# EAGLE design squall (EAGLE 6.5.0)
AUTHOR: Brad Campbell; REV: A; TITLE: Squall

## Sheet 1 of 2: nRF51822
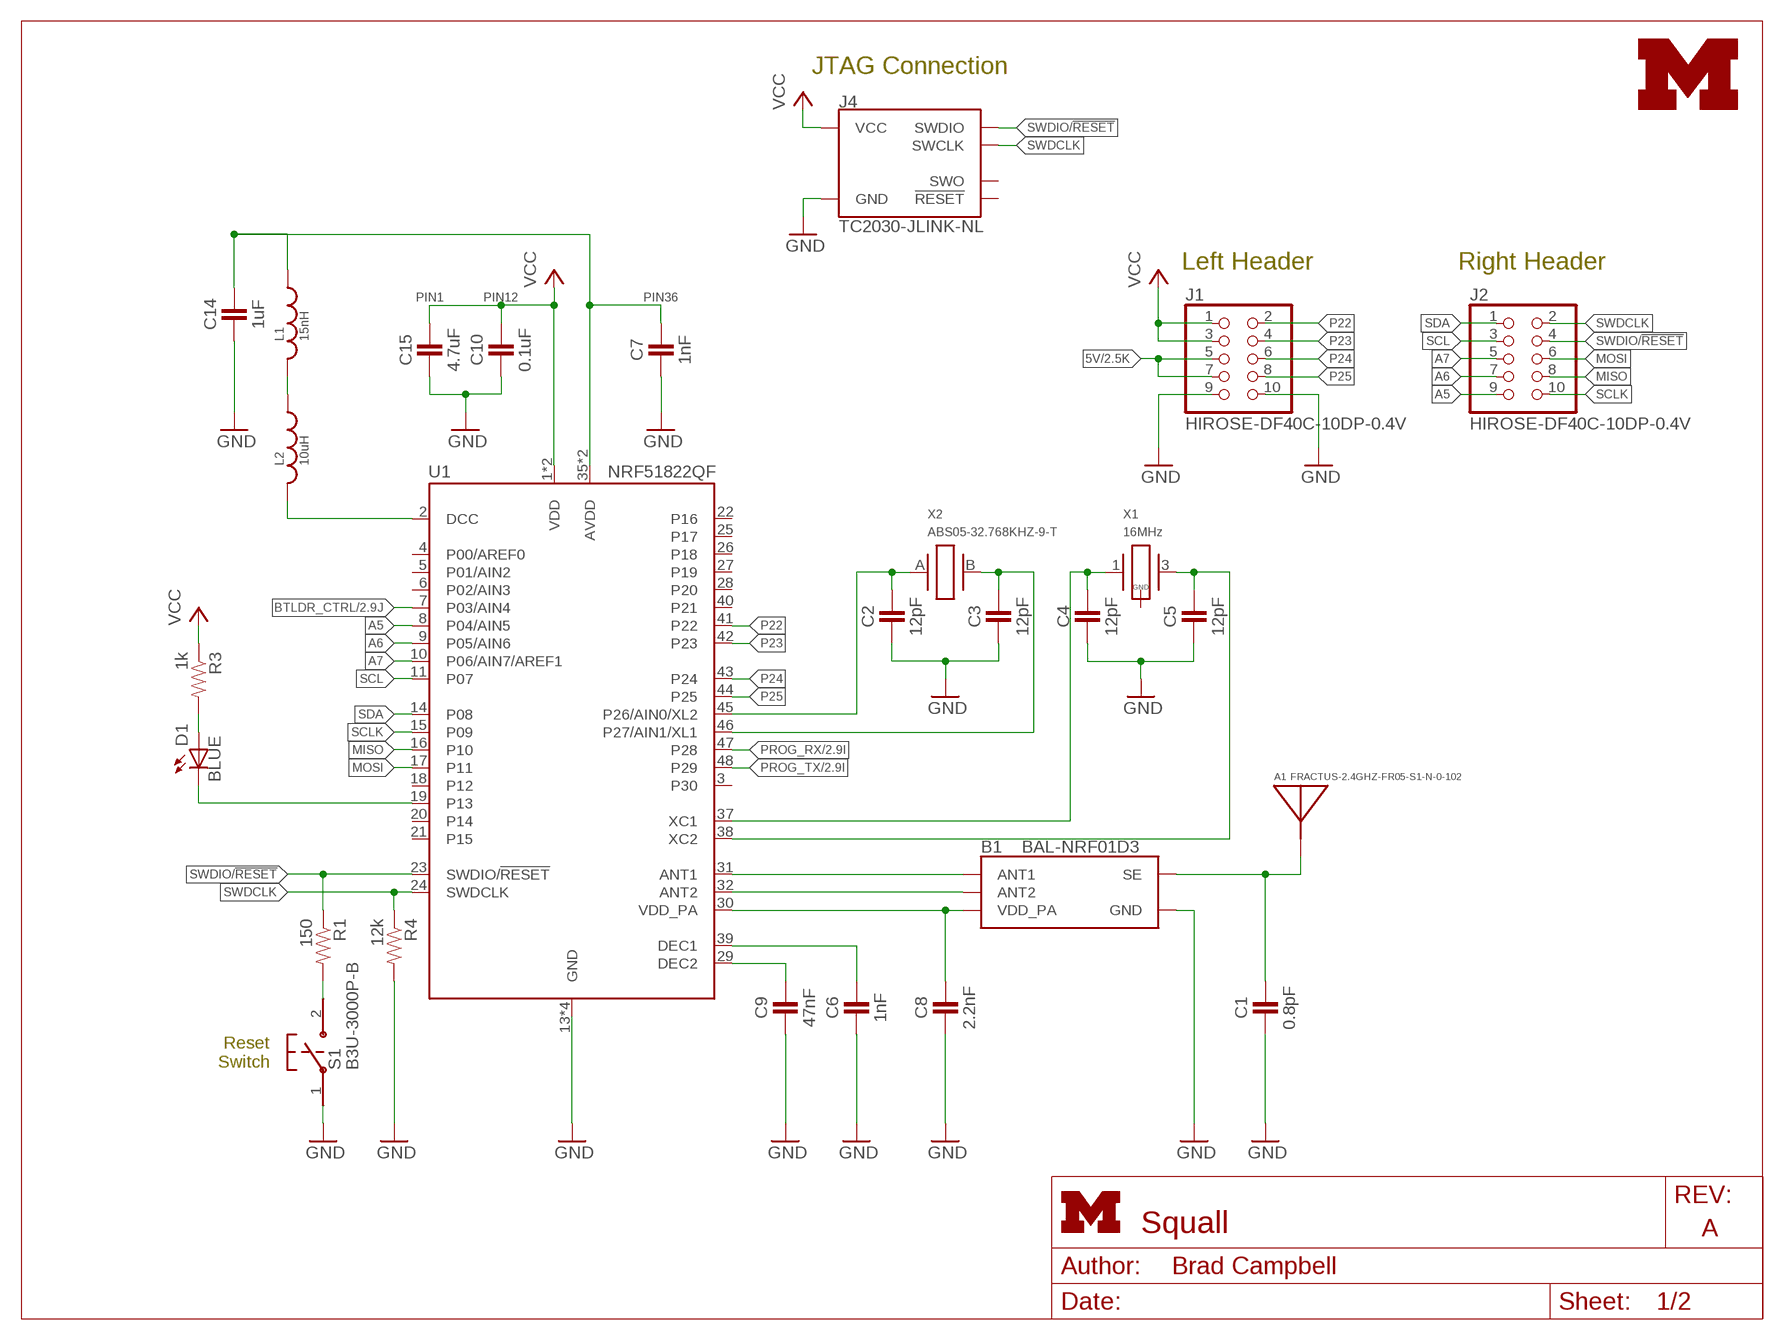
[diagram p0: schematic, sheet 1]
FRAME1 (LETTER_L): HEIGHT: 8.5in; WIDTH: 11in

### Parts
A1  FRACTUS-2.4GHZ-FR05-S1-N-0-102  [FRACTUS-ANTENNA-FR05-S1-N-0-102]
B1  BAL-NRF01D3  [BAL-NRF01D3]
C1  0.8pF  CAPACITOR  [0402_CAP]
C2  12pF  CAPACITOR  [0402_CAP]
C3  12pF  CAPACITOR  [0402_CAP]
C4  12pF  CAPACITOR  [0402_CAP]
C5  12pF  CAPACITOR  [0402_CAP]
C6  1nF  CAPACITOR  [0402_CAP]
C7  1nF  CAPACITOR  [0402_CAP]
C8  2.2nF  CAPACITOR  [0402_CAP]
C9  47nF  CAPACITOR  [0402_CAP]
C10  0.1uF  CAPACITOR  [0402_CAP]
C14  1uF  CAPACITOR  [0402_CAP]
C15  4.7uF  CAPACITOR  [0402_CAP]
D1  BLUE  LED0603  [LED-0603]
J1  HIROSE-DF40C-10DP-0.4V  [2X5/SMD/0.4MM]
J2  HIROSE-DF40C-10DP-0.4V  [2X5/SMD/0.4MM]
J4  TC2030-JLINK-NL  [TC2030-IDC-NL]
L1  15nH  INDUCTOR0402  [0402_CAP]
L2  10uH  INDUCTOR0603  [0603_CAP]
LOGO1  UMICH_SOLID_TINY  [UMICH_SOLID_50MIL]
R1  150  RESISTOR  [0402_RES]
R3  1k  RESISTOR  [0402_RES]
R4  12k  RESISTOR  [0402_RES]
S1  B3U-3000P-B  [B3U-3000P-B]
U1  NRF51822QF  [QFN-48-6MM]
X1  16MHz  TXC-8Y  [TXC-8Y]
X2  ABS05-32.768KHZ-9-T  [ABS05]

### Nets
5V: J1.5 J1.7 ; also sheet 2
A0: C2.1 U1.45(P26/AIN0/XL2) X2.A
A1: C3.1 U1.46(P27/AIN1/XL1) X2.B
A5: J2.9 U1.8(P04/AIN5)
A6: J2.7 U1.9(P05/AIN6)
A7: J2.5 U1.10(P06/AIN7/AREF1)
AVDD: C7.1 C14.1 L1.1 U1.35(AVDD) U1.36(AVDD)
BTLDR_CTRL: U1.7(P03/AIN4) ; also sheet 2
DCC: L2.2 U1.2(DCC)
GND: B1.GND C1.2 C2.2 C3.2 C4.2 C5.2 C6.2 C7.2 C8.2 C9.2 C10.2 C14.2 C15.2 J1.9 J1.10 J4.5(GND) R4.2 S1.1 U1.13(GND) U1.33(GND) U1.34(GND) U1.GND ; also sheet 2
MISO: J2.8 U1.16(P10)
MOSI: J2.6 U1.17(P11)
N$5: B1.ANT1 U1.31(ANT1)
N$6: B1.ANT2 U1.32(ANT2)
N$7: D1.C U1.19(P13)
N$8: R1.2 S1.2
N$11: A1.1(ANTENNA) B1.SE C1.1
N$14: L1.2 L2.1
N$16: C4.1 U1.37(XC1) X1.1
N$17: C5.1 U1.38(XC2) X1.3
N$18: C6.1 U1.39(DEC1)
N$19: C9.1 U1.29(DEC2)
N$23: D1.A R3.2
P22: J1.2 U1.41(P22)
P23: J1.4 U1.42(P23)
P24: J1.6 U1.43(P24)
P25: J1.8 U1.44(P25)
PROG_RX: U1.47(P28) ; also sheet 2
PROG_TX: U1.48(P29) ; also sheet 2
SCL: J2.3 U1.11(P07)
SCLK: J2.10 U1.15(P09)
SDA: J2.1 U1.14(P08)
SWDCLK: J2.2 J4.4(SWCLK) R4.1 U1.24(SWDCLK)
SWDIO/!RESET: J2.4 J4.2(SWDIO) R1.1 U1.23(SWDIO/!RESET)
VCC: C10.1 C15.1 J1.1 J1.3 J4.1(VCC) R3.1 U1.1(VDD) U1.12(VDD) ; also sheet 2
VDD_PA: B1.VCC(VDD_PA) C8.1 U1.30(VDD_PA)
Unconnected: J4.3(!RESET) J4.6(SWO) U1.3(P30) U1.4(P00/AREF0) U1.5(P01/AIN2) U1.6(P02/AIN3) U1.18(P12) U1.20(P14) U1.21(P15) U1.22(P16) U1.25(P17) U1.26(P18) U1.27(P19) U1.28(P20) U1.40(P21) X1.2(GND) X1.4(GND)

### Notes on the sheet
- JTAG Connection
- Left Header | Right Header
- PIN1 | PIN12 | PIN36
- Reset
  Switch

## Sheet 2 of 2: Programmer and Batteries
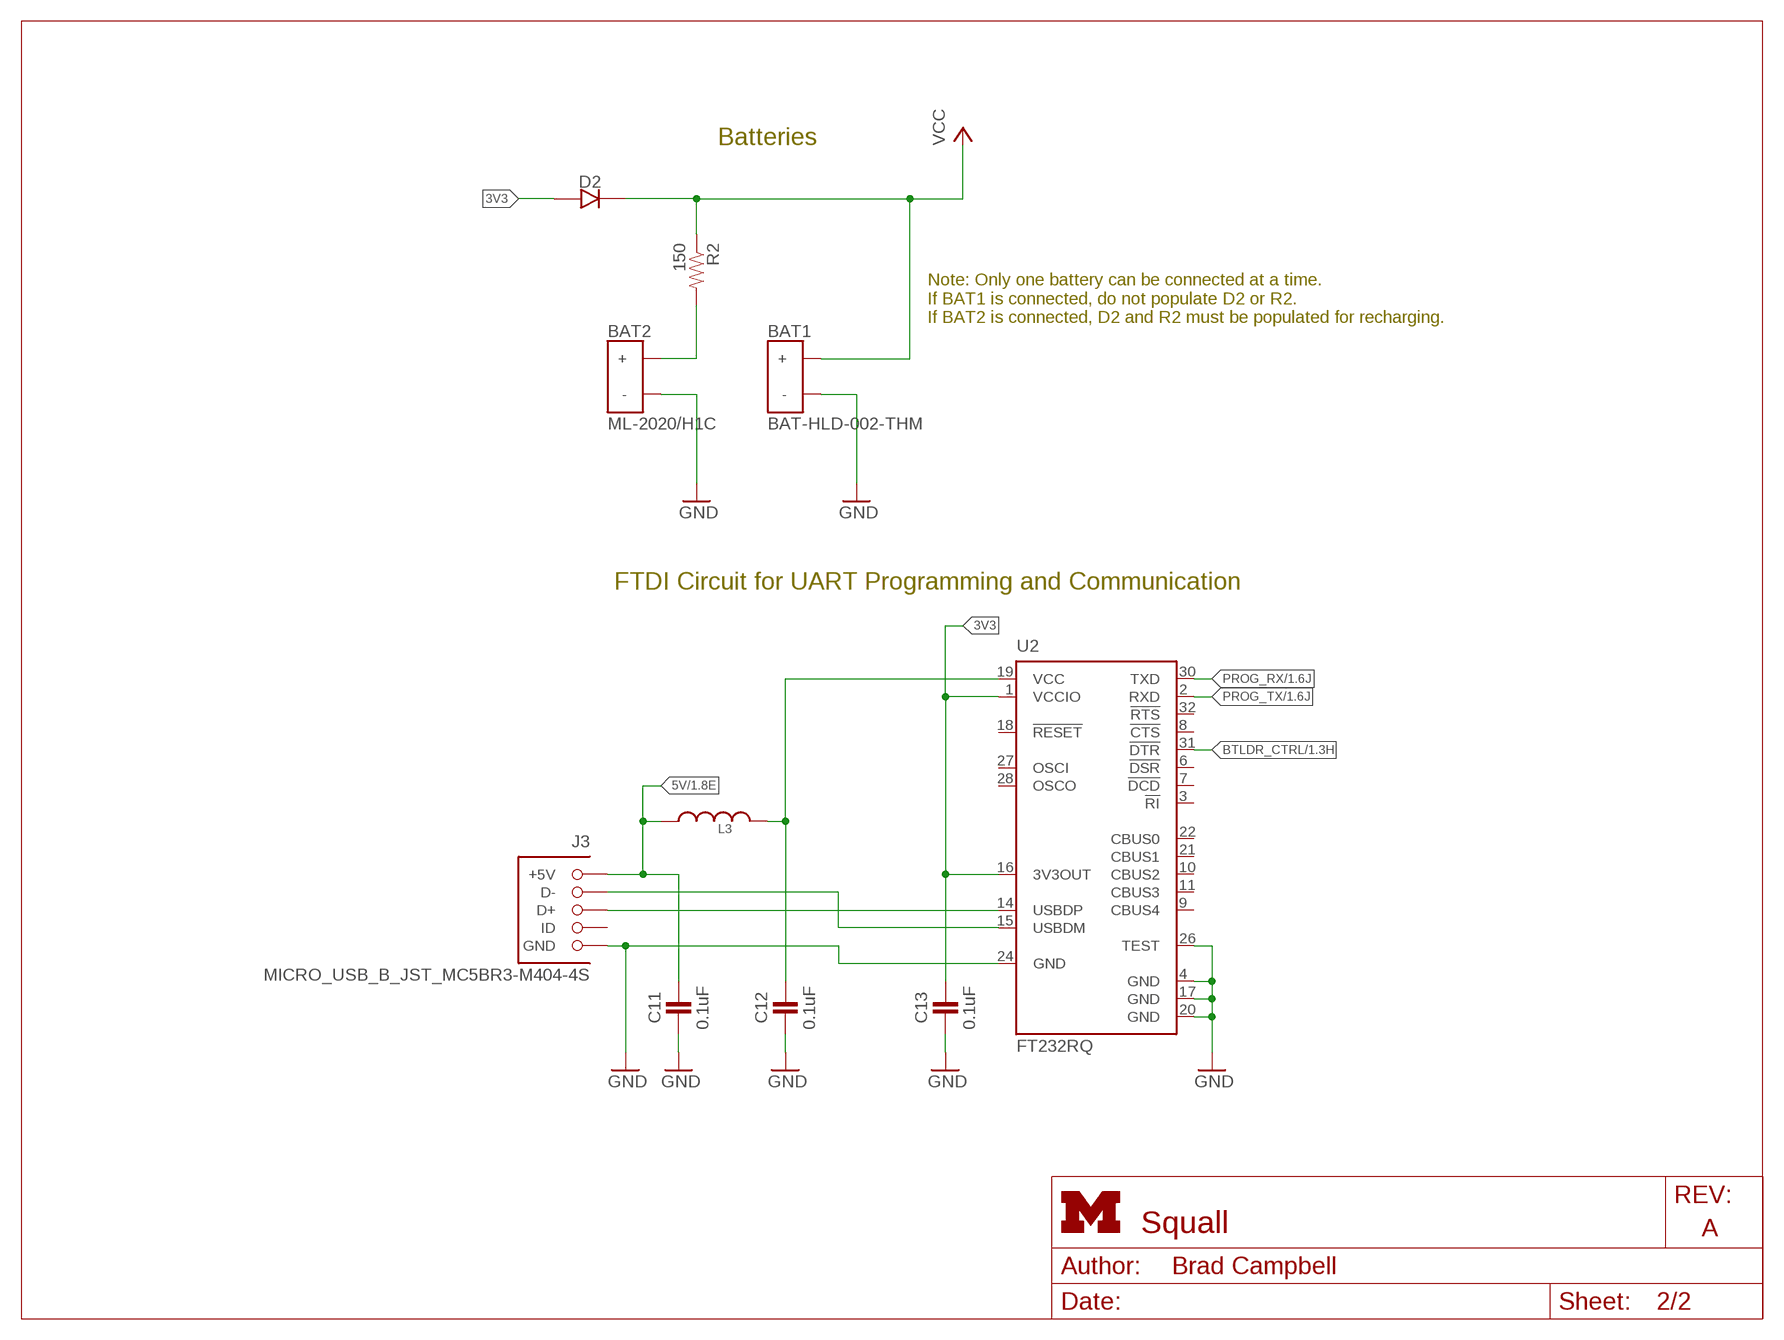
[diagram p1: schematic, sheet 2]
FRAME2 (LETTER_L): HEIGHT: 8.5in; WIDTH: 11in

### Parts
BAT1  BAT-HLD-002-THM  [BAT-HLD-002-THM]
BAT2  ML-2020/H1C  [ML-2020/H1C]
C11  0.1uF  CAPACITOR  [0402_CAP]
C12  0.1uF  CAPACITOR  [0402_CAP]
C13  0.1uF  CAPACITOR  [0402_CAP]
D2  DIODE  [0402_DIODE]
J3  MICRO_USB_B_JST_MC5BR3-M404-4S  [USB_MICRO_B-JST-MC5BR3-M404-4S-TB]
L3  INDUCTOR0402  [0402_CAP]
R2  150  RESISTOR  [0402_RES]
U2  FT232RQ  [QFN32]

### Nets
3V3: C13.1 D2.ANODE U2.1(VCCIO) U2.16(3V3OUT)
5V: C11.1 J3.1(+5V) L3.1 ; also sheet 1
BTLDR_CTRL: U2.31(!DTR) ; also sheet 1
FTDI_VCC: C12.1 L3.2 U2.19(VCC)
GND: BAT1.GND(-) BAT2.NEG(-) C11.2 C12.2 C13.2 J3.5(GND) U2.4(GND) U2.17(GND) U2.20(GND) U2.24(GND) U2.26(TEST) ; also sheet 1
N$1: BAT2.POS(+) R2.2
N$26: J3.3(D+) U2.14(USBDP)
N$27: J3.2(D-) U2.15(USBDM)
PROG_RX: U2.30(TXD) ; also sheet 1
PROG_TX: U2.2(RXD) ; also sheet 1
VCC: BAT1.POS1(+) BAT1.POS2(+) BAT1.POS3(+) BAT1.POS4(+) D2.CATHODE R2.1 ; also sheet 1
Unconnected: J3.4(ID) U2.3(!RI) U2.6(!DSR) U2.7(!DCD) U2.8(!CTS) U2.9(CBUS4) U2.10(CBUS2) U2.11(CBUS3) U2.18(!RESET) U2.21(CBUS1) U2.22(CBUS0) U2.27(OSCI) U2.28(OSCO) U2.32(!RTS)

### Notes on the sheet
- Batteries
- Note: Only one battery can be connected at a time.
  If BAT1 is connected, do not populate D2 or R2.
  If BAT2 is connected, D2 and R2 must be populated for recharging.
- FTDI Circuit for UART Programming and Communication

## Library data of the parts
A1 = chips:FRACTUS-2.4GHZ-FR05-S1-N-0-102: Fractus Compact Reach XtendTM chip antenna is engineered specifically for Bluetooth,; RICHARDSON_RFPD: FR05-S1-N-0102B
B1 = chips:BAL-NRF01D3: 50 ohm nominal input / conjugate match balun to nRF51422-QFAA, nRF24LE1, nRF51822-QFAA/AB, with integrated harmonic filter; DIGIKEY: 497-13637-1-ND; MOUSER: 511-BAL-NRF01D3
BAT1 = batteries:BAT-HLD-002-THM: RETAINER BATT CR2016 PC PINS; DIGIKEY: BAT-HLD-002-THM-ND; MOUSER: 712-BAT-HLD-002-THM
BAT2 = batteries:ML-2020/H1C: BATT LITH COIN 3V RECHARGE PINS 45mAh; DIGIKEY: P047-ND; MOUSER: 658-ML-2020/H1CN
C1 = passives:CAPACITOR: 0402 Capacitor; DIGIKEY: 490-6269-1-ND
C2-C5 = passives:CAPACITOR: 0402 Capacitor; DIGIKEY: 490-6197-1-ND
C6 C7 = passives:CAPACITOR: 0402 Capacitor; DIGIKEY: 490-1303-1-ND
C8 = passives:CAPACITOR: 0402 Capacitor; DIGIKEY: 490-5419-1-ND
C9 = passives:CAPACITOR: 0402 Capacitor; DIGIKEY: 445-1264-1-ND
C10 = passives:CAPACITOR: 0402 Capacitor; DIGIKEY: 445-4952-1-ND
C11-C13 = passives:CAPACITOR: 0402 Capacitor; DIGIKEY: 490-1318-6-ND
C14 = passives:CAPACITOR: 0402 Capacitor; DIGIKEY: 1276-1513-1-ND
C15 = passives:CAPACITOR: 0402 Capacitor; DIGIKEY: 445-5947-1-ND
D1 = SparkFun-LED:LED: LEDs
D2 = passives:DIODE; DIGIKEY: 641-1271-1-ND; MOUSER: 750-CDBQR0130L
J1 J2 = headers:HIROSE-DF40C-10DP-0.4V: DF40 Series Header - 0.4MM Pitch; DIGIKEY: H11616CT-ND; MOUSER: 798-DF40C10DP0.4V51; NEWARK: 68X2585
J3 = connector:MICRO_USB_B_JST_MC5BR3-M404-4S: Micro USB B mid mount; DIGIKEY: 455-2567-2-ND; MOUSER: 53X3655
J4 = connector:TC2030-JLINK
L1 = passives:INDUCTOR; DIGIKEY: 587-1521-1-ND
L2 = passives:INDUCTOR; DIGIKEY: 490-4025-1-ND
L3 = passives:INDUCTOR; DIGIKEY: 445-2979-1-ND
LOGO1 = logos:UMICH_SOLID
R1 R2 = passives:RESISTOR: Resistor; DIGIKEY: RHM150CDCT-ND
R3 = passives:RESISTOR: Resistor; DIGIKEY: RHM1.0KCECT-ND
R4 = passives:RESISTOR: Resistor; DIGIKEY: RHM12.0KCDCT-ND
S1 = switches:B3U; DIGIKEY: SW1256CT-ND
U1 = chips:NRF51822: Multiprotocol Bluetooth® 4.0 low energy/2.4 GHz RF SoC; DIGIKEY: 1490-1032-1-ND; MOUSER: 949-NRF51822-QFAB-R7
U2 = ftdichip:FT232R: Source: http://www.ftdichip.com/Documents/DataSheets/DS_FT232R_v104.pdf; MPN: FT232RQ; OC_FARNELL: 1146033; OC_NEWARK: 91K9919
X1 = crystals:TXC-8Y: 2mmx1.6mm SMD Crystal; DIGIKEY: 887-2003-1-ND
X2 = crystals:ABS05-32.768KHZ: 32.768kHz Crystal; DIGIKEY: 535-11897-1-ND

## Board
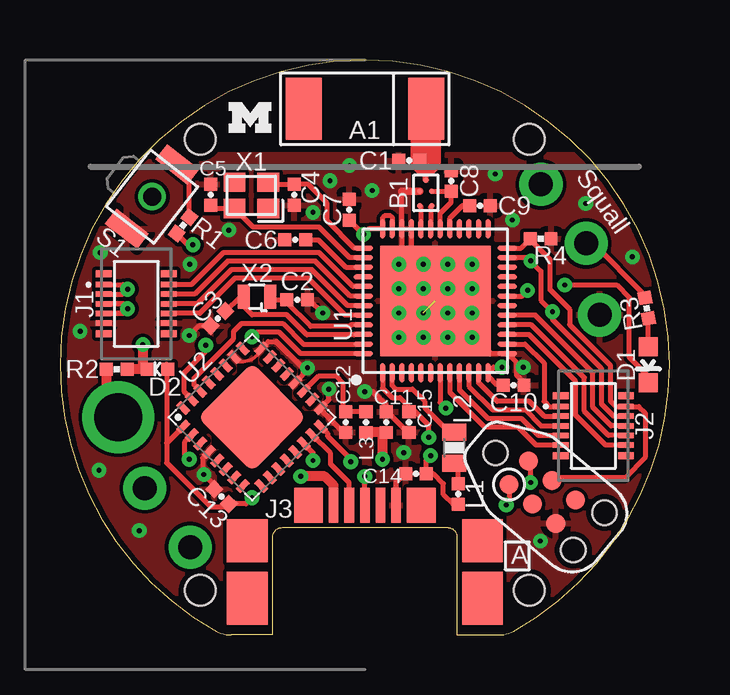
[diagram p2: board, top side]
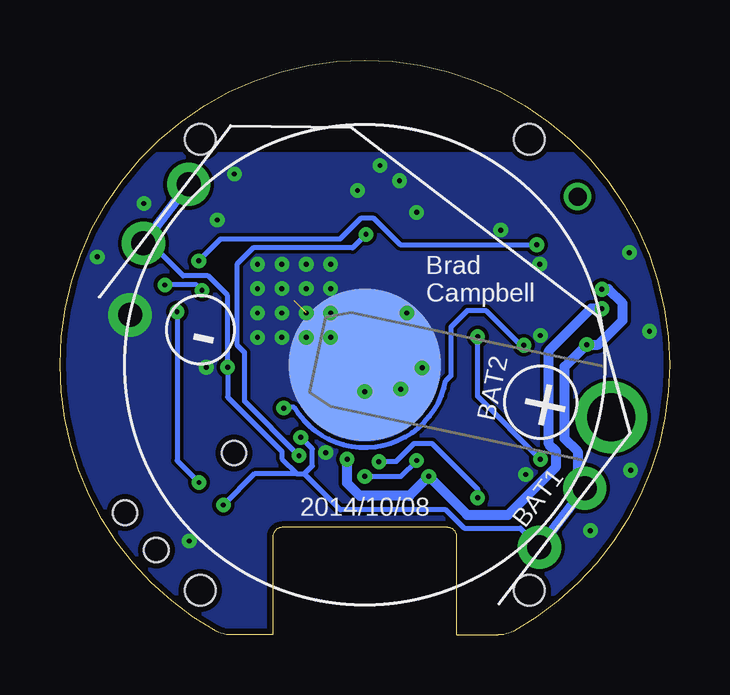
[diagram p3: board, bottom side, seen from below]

Size 25.4 x 23.95 mm. Coordinates in mm from the lower left corner, seen from the top.
Outline: 8.87,0 7.14,0 arc-29 6.5,0.15 arc-61 0,11.25 arc-90 12.7,23.95 arc-90 25.4,11.25 arc-61 18.9,0.15 arc-29 18.26,0 16.54,0
Copper layers (1*16): Top 0.0178mm / dielectric 59mil / Bottom 0.0178mm
Design rules "sunstone-2lyr_v1.0.0.3 *": minimum track width 6mil, minimum drill 14mil, track to track 6mil, track to pad 6mil, pad to pad 6mil, via to via 6mil, smd to smd 6mil, copper to edge 10mil, drill to drill 16mil, minimum pad ring 8mil, minimum via ring 8mil, stop-mask expansion 3mil, vias tented up to drill 50mil, thermal gap 10mil
Holes 1.27 mm at 19.56,20.65 5.84,20.65 5.84,1.85 19.56,1.85

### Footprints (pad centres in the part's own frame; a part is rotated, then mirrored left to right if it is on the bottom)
FRACTUS-ANTENNA-FR05-S1-N-0-102 = smd 1.5 x 2.6: 1 -2.55,0; 2 2.55,0
BAL-NRF01D3 = smd 0.22 x 0.22: ANT1 -0.537,-0.25; ANT2 -0.537,0.25; GND 0.069,0.25; SE 0.537,0; VCC 0.069,-0.25
BAT-HLD-002-THM = smd 6.35 x 6.35: GND 0,0 | drill 1 pad 1.8: POS1 -10.4,1.5; POS2 -10.4,-1.6; POS3 10.4,1.5; POS4 10.4,-1.6
ML-2020/H1C = drill 1 pad 1.8: NEG -10,0 | drill 2 pad 2.3: POS 10.5,0
0402_CAP = smd 0.536 x 0.546: 1 -0.433,0; 2 0.433,0
LED-0603 = smd 0.8 x 0.8: A 0,-0.75; C 0,0.75
0402_DIODE = smd 0.536 x 0.546: ANODE -0.433,0; CATHODE 0.433,0
2X5/SMD/0.4MM = smd 0.66 x 0.23: 1 -1.355,0.8; 2 1.355,0.8; 3 -1.355,0.4; 4 1.355,0.4; 5 -1.355,0; 6 1.355,0; 7 -1.355,-0.4; 8 1.355,-0.4; 9 -1.355,-0.8; 10 1.355,-0.8 | smd 0.66 x 0.3: A -1.355,1.25; B 1.355,1.25; C -1.355,-1.25; D 1.355,-1.25
USB_MICRO_B-JST-MC5BR3-M404-4S-TB = smd 0.4 x 1.45: 1 -1.3,3.875; 2 -0.65,3.875; 3 0,3.875; 4 0.65,3.875; 5 1.3,3.875 | smd 1.7 x 2.2: P$1 -4.9,0; P$2 4.9,0 | smd 1.7 x 1.8: P$3 -4.9,2.4; P$4 4.9,2.4 | smd 1.2 x 1.45: P$5 -2.35,3.875; P$6 2.35,3.875
TC2030-IDC-NL = smd 0.787 x 0.787: 1 -1.27,-0.635; 2 -1.27,0.635; 3 0,-0.635; 4 0,0.635; 5 1.27,-0.635; 6 1.27,0.635 | hole 1.016: -2.54,0; 2.54,1.016; 2.54,-1.016
0603_CAP = smd 0.7 x 1: 1 -0.65,0; 2 0.65,0
0402_RES = smd 0.536 x 0.546: 1 -0.433,0; 2 0.433,0
B3U-3000P-B = smd 0.8 x 1.7: 1 -1.7,0; 2 1.7,0 | drill 0.75: P$1 0,0
QFN-48-6MM = smd 0.8 x 0.203: 1 -3,2.2; 2 -3,1.8; 3 -3,1.4; 4 -3,1; 5 -3,0.6; 6 -3,0.2; 7 -3,-0.2; 8 -3,-0.6; 9 -3,-1; 10 -3,-1.4; 11 -3,-1.8; 12 -3,-2.2; 25 3,-2.2; 26 3,-1.8; 27 3,-1.4; 28 3,-1; 29 3,-0.6; 30 3,-0.2; 31 3,0.2; 32 3,0.6; 33 3,1; 34 3,1.4; 35 3,1.8; 36 3,2.2 | smd 0.203 x 0.8: 13 -2.2,-3; 14 -1.8,-3; 15 -1.4,-3; 16 -1,-3; 17 -0.6,-3; 18 -0.2,-3; 19 0.2,-3; 20 0.6,-3; 21 1,-3; 22 1.4,-3; 23 1.8,-3; 24 2.2,-3; 37 2.2,3; 38 1.8,3; 39 1.4,3; 40 1,3; 41 0.6,3; 42 0.2,3; 43 -0.2,3; 44 -0.6,3; 45 -1,3; 46 -1.4,3; 47 -1.8,3; 48 -2.2,3 | smd 4.6 x 4.6: GND 0,0
QFN32 = smd 0.6 x 0.3: 1 -2.3,1.75; 2 -2.3,1.25; 3 -2.3,0.75; 4 -2.3,0.25; 5 -2.3,-0.25; 6 -2.3,-0.75; 7 -2.3,-1.25; 8 -2.3,-1.75; 17 2.3,-1.75; 18 2.3,-1.25; 19 2.3,-0.75; 20 2.3,-0.25; 21 2.3,0.25; 22 2.3,0.75; 23 2.3,1.25; 24 2.3,1.75 | smd 0.3 x 0.6: 9 -1.75,-2.3; 10 -1.25,-2.3; 11 -0.75,-2.3; 12 -0.25,-2.3; 13 0.25,-2.3; 14 0.75,-2.3; 15 1.25,-2.3; 16 1.75,-2.3; 25 1.75,2.3; 26 1.25,2.3; 27 0.75,2.3; 28 0.25,2.3; 29 -0.25,2.3; 30 -0.75,2.3; 31 -1.25,2.3; 32 -1.75,2.3 | smd 3.2 x 3.2: EXP 0,0
TXC-8Y = smd 0.9 x 0.8: 1 -0.7,-0.55; 2 0.7,-0.55; 3 0.7,0.55; 4 -0.7,0.55
ABS05 = smd 0.5 x 1: A -0.55,0; B 0.55,0

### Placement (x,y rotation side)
A1  12.7,21.92 180 top
B1  15.24,18.41 90 top
BAT1  12.7,11.25 322.5 bottom
BAT2  12.7,11.25 348 bottom
C1  14.55,19.76 180 top
C2  9.88,13.97 0 top
C3  6.58,13.18 225 top
C4  9.75,18.34 270 top
C5  6.27,18.34 90 top
C6  9.8,16.46 180 top
C7  12.05,17.71 90 top
C8  16.3,18.91 90 top
C9  17.5,17.88 0 top
C10  18.9,10.41 0 top
C11  13.59,8.86 90 top
C12  11.91,8.86 270 top
C13  6.73,5.77 135 top
C14  14.83,6.71 180 top
C15  14.54,8.86 270 top
D1  24.51,11.25 180 top
D2  4.06,11.07 180 top
J1  3.17,13.79 0 top
J2  22.23,8.71 0 top
J3  12.7,1.52 0 top
J4  20.09,5.94 320 top
L1  16.59,5.87 90 top
L2  16.43,7.8 90 top
L3  12.75,8.86 90 top
LOGO1  7.92,21.56 0 top
R1  5.13,17.06 52 top
R2  2.36,11.07 180 top
R3  24.45,13.61 280 top
R4  20.03,16.5 0 top
S1  3.84,18.26 52 top
U1  15.64,13.92 90 top
U2  8,9.07 45 top
X1  7.98,18.31 180 top
X2  8.2,14.1 180 top

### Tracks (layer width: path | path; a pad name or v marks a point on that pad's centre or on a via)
3V3  (via drill 0.2)
  Top 0.203: 5.14,8.67 U2.1 4.45,7.99 | U2.16 11.15,8.39 11.15,8.28 12.12,7.32 v12.12,7.21 | 4.45,7.99 4.45,11.28 D2.ANODE | 4.45,7.99 4.45,7.16 6.27,5.33 6.91,5.33 C13.1 7.75,5.46 v8,5.72
  Bottom 0.203: v8,5.72 8,6.07 9.91,7.98 10.64,7.98 11.4,7.21 v12.12,7.21
5V  (via drill 0.2)
  Top 0.229: J1.5 2.62,13.79 v2.82,13.59 2.62,13.39 J1.7
  Top 0.406: J3.1 11.4,6.23 11.02,6.6 v10.03,6.6 | L3.1 C11.1 13.44,8.28 v13.44,7.32
  Bottom 0.406: v2.82,13.59 3.28,13.59 5.03,11.84 5.03,7.95 4.72,7.65 4.72,7.01 6.73,5 8.43,5 v10.03,6.6 10.85,5.79 12.9,5.79 13.44,6.32 v13.44,7.32
A0
  Top 0.203: U1.45 12.13,12.92 12.06,12.85 10.44,12.85 9.45,13.84 C2.1 8.88,13.97 X2.A
A1
  Top 0.203: U1.46 12.26,12.52 12.24,12.5 10.29,12.5 9.45,13.34 8,13.34 7.65,13.68 X2.B 7.52,14.1 C3.1
A5
  Top 0.203: U1.8 16.24,10.1 17.68,8.66 19.07,8.66 19.82,7.91 J2.9
A6
  Top 0.203: U1.9 16.64,10.21 17.83,9.02 19.23,9.02 19.93,8.31 J2.7
A7
  Top 0.203: U1.10 17.04,10.37 18.03,9.37 19.38,9.37 20.04,8.71 J2.5
AVDD  (via drill 0.2)
  Top 0.203: U1.35 13.84,17.4 13.74,17.48 13.54,17.48 13.44,17.38 U1.36 12.88,16.92 v12.65,16.69 12.59,16.74 C7.1 | L1.1 16.38,5.43 15.98,5.84 15.98,6.3 15.57,6.71 C14.1 15.27,7.29 v15.44,7.47
  Bottom 0.203: v15.44,7.47 17.7,9.73 17.7,11.76 18.01,12.07 18.01,15.47 17.35,16.13 13.21,16.13 v12.65,16.69
BTLDR_CTRL  (via drill 0.2)
  Top 0.203: U2.31 5.18,10.12 5.18,10.92 6.07,11.81 v6.07,12.07 | U1.7 15.84,9.69 v16.08,9.45
  Bottom 0.203: v16.08,9.45 16.05,9.47 15.65,9.47 arc-138 9.32,10.59 9.12,10.8 9.12,12.83 8.43,13.51 7.64,13.51 6.2,12.07 v6.07,12.07
DCC
  Top 0.203: U1.2 13.84,10.39 13.99,10.24 14.68,10.24 15.21,9.7 15.21,9.45 16.22,8.45 L2.2
FTDI_VCC
  Top 0.203: U2.19 10.79,10.8 11.48,10.8 11.79,10.49 11.79,9.42 C12.1 L3.2
GND  (via drill 0.2)  (1 unrouted)
  Top 0.152: 8.3,11.93 U2.24 arc-67 7.56,11.38 7.46,11.38 U2.26
  Top 0.203: U2.24 8.68,12.22 9.02,12.22 10.11,11.13 | 10.11,11.13 10.11,10.82 U2.20 | C12.2 11.81,8.43 10.87,9.38 U2.17 11.2,9.79 v11.2,10.24 | v10.31,11.13 10.11,11.13 | C15.2 14.48,8.43 13.97,8.97 13.64,9.3 C11.2 13.59,9.58 13.03,10.13 v12.7,10.13 | U2.4 5.94,7.36 5.94,6.73 v5.99,6.68 6.42,6.25 C13.2 | C10.2 19.41,10.44 19.02,10.82 19.02,11.33 U1.13 17.98,11.72 v17.17,12.4 | J3.5 14,6.38 C14.2 | 14.24,18.48 U1.34 14.24,15.69 v14.12,15.44 14.64,16.09 U1.33 | v15.14,12.4 v14.12,12.4 | C2.2 10.39,13.97 v10.95,13.41 | C3.2 5.79,12.88 v5.38,12.47
  Top 0.305: B1.GND 14.24,18.48
  Bottom 0.203: v12.7,10.13 12.14,9.58 10.34,9.58
  other vias: 14.33,7.59 15.14,14.43 16.15,14.43 17.17,14.43 14.12,14.43 15.14,15.44 16.15,15.44 17.17,15.44 17.17,13.41 16.15,13.41 14.12,13.41 15.14,13.41 16.15,12.4 11.25,18.92 13,18.52 10.54,17.6 18.85,17.28 3.3,4.34 21.91,17.97 20.02,3.91 19.3,11.15 7.04,16.87 5.41,15.44 1.68,15.93 18.14,19.2 12.06,19.56 23.85,15.75 1.63,6.86 0.84,12.65
  pour Top: -1.27,20.02 14.5,20.02 14.5,16.64 16.1,16.64 16.1,20.02 26.67,20.02 26.67,-2.72 -1.27,-2.72
  pour Bottom (no thermals): 26.67,-2.72 26.67,20.02 -1.27,20.02 -1.27,-2.72
MISO
  Top 0.203: U1.16 19.64,12.92 21.84,10.72 21.84,9.32 22.85,8.31 J2.8
MOSI
  Top 0.203: U1.17 19.8,13.32 22.2,10.92 22.2,9.47 22.96,8.71 J2.6
N$1
  Top 0.406: R2.2 1.93,9.57 BAT2.POS
N$5
  Top 0.203: B1.ANT1 15.44,17.83 U1.31
N$6
  Top 0.203: B1.ANT2 15.04,17.83 U1.32
N$7  (via drill 0.2)
  Top 0.203: U1.19 19.25,14.12 v19.48,14.35 | v21.03,14.58 23.19,14.58 23.72,14.05 23.72,11.56 24.51,10.77 D1.C
  Bottom 0.203: v21.03,14.58 19.71,14.58 v19.48,14.35
N$8
  Top 0.203: R1.2 5.39,19.09 S1.2
N$11
  Top 0.203: 15.24,19.29 15.24,19.76
  Top 0.254: B1.SE 15.24,19.29
  Top 0.762: 15.24,19.76 C1.1 | 15.24,21.91 A1.1
  Top 1.27: 15.24,19.76 15.24,21.91
N$14
  Top 0.203: L1.2 16.59,7 L2.1
N$16
  Top 0.203: U1.37 12.25,16.12 11.12,17.25 11.12,17.98 10.34,18.77 C4.1 8.31,18.77 X1.1
N$17
  Top 0.203: U1.38 12.07,15.72 10.79,16.99 8.05,16.99 X1.3 6.42,17.76 C5.1
N$18
  Top 0.203: C6.1 10.77,16.46 11.91,15.32 U1.39
N$19
  Top 0.203: U1.29 16.24,17.36 16.76,17.88 C9.1
N$23
  Top 0.203: D1.A 24.51,13.18 R3.2
N$26  (via drill 0.2)
  Top 0.203: J3.3 v12.7,6.6 | U2.14 10.54,7.59 v10.54,7.26
  Bottom 0.203: v12.7,6.6 11.2,6.6 v10.54,7.26
N$27
  Top 0.203: J3.2 12.05,6.34 11.28,7.11 11.28,7.56 U2.15
P22
  Top 0.203: U1.41 12.2,14.52 10.79,15.93 6.81,15.93 5.47,14.59 J1.2
P23
  Top 0.203: U1.42 12.1,14.12 10.64,15.57 6.99,15.57 5.61,14.19 J1.4
P24
  Top 0.203: U1.43 11.99,13.72 10.49,15.21 7.14,15.21 5.71,13.79 J1.6
P25
  Top 0.203: U1.44 11.88,13.32 10.34,14.86 7.29,14.86 5.82,13.39 J1.8
PROG_RX
  Top 0.203: U1.47 10.13,12.12 9.27,12.98 7.57,12.98 7.24,12.65 7.24,12.34 5.59,10.69 5.59,10.42 U2.30
PROG_TX  (via drill 0.2)
  Top 0.203: U1.48 10.02,11.72 9.14,12.6 8.18,12.6 v8,12.42 | U2.2 5.18,8.02 5.18,7.52 v5.38,7.32
  Bottom 0.203: v8,12.42 8,9.93 v5.38,7.32
SCL
  Top 0.203: U1.11 17.44,10.5 18.21,9.73 19.56,9.73 20.17,9.11 J2.3
SCLK
  Top 0.203: U1.15 19.54,12.52 21.46,10.59 21.46,9.17 22.72,7.91 J2.10
SDA
  Top 0.203: U1.14 19.38,12.12 20.17,11.33 20.17,9.73 20.38,9.51 J2.1
SWDCLK
  Top 0.203: J4.4 20.62,6.55 23.55,6.55 24.38,7.39 24.38,9.25 24.12,9.51 J2.2 23.18,9.51 22.94,9.75 22.94,11.23 21.23,12.93 21.23,13.56 20.42,14.38 20.42,15.63 19.59,16.46 R4.1 19.22,16.12 U1.24
SWDIO/!RESET  (via drill 0.2)
  Top 0.203: 19.05,15.72 U1.23 19.48,15.72 v19.62,15.58 20.04,15.16 20.04,13.94 v20.52,13.46 20.52,13.13 22.55,11.1 22.55,9.63 23.07,9.11 J2.4 | v19.61,6.35 19.61,7.16 J4.2 | v5.54,16.26 5.33,16.26 R1.1
  Bottom 0.203: v20.52,13.46 20.52,7.26 v19.61,6.35 | v5.54,16.26 11.23,16.26 12.32,17.35 12.88,17.35 13.74,16.48 18.71,16.48 v19.62,15.58
VCC  (via drill 0.2)
  Top 0.203: U1.1 13.44,10.28 13.84,9.88 14.17,9.88 14.54,9.51 C15.1 14.81,9.3 15.37,8.74 v15.37,8.23 | U1.12 17.84,10.81 | J1.1 2.63,14.59 v2.82,14.4 2.61,14.19 J1.3 | C10.1 18.22,10.41 17.84,10.79 U1.12 | U1.12 18.07,11.15 v18.41,11.15 | J4.1 18.71,5.53 v18.59,5.41 | R3.1 24.37,14.16 22.22,16.31 BAT1.POS2
  Top 0.406: R2.1 D2.CATHODE 3.45,11.25 v3.45,12.09
  Bottom 0.203: 15.21,6.71 14.88,7.04 14.88,7.75 v15.37,8.23 | 15.21,6.71 13.72,5.21 9.32,5.21 8.56,4.45 6.22,4.45 BAT1.POS4 | 15.52,6.71 17.3,6.71 v18.59,5.41 | 15.52,6.71 16.15,7.34 16.15,7.65 18.41,9.91 v18.41,11.15 18.41,14.15 19.23,14.96 20.27,14.96 21.62,16.31 BAT1.POS2 | 15.52,6.71 15.21,6.71
  Bottom 0.406: v2.82,14.4 2.55,14.4 1.96,13.81 1.96,13.11 2.97,12.09 v3.45,12.09 4.37,11.18 4.37,8.18 3.83,7.65 3.83,6.41 BAT1.POS3 BAT1.POS4 | BAT1.POS2 BAT1.POS1
VDD_PA
  Top 0.203: U1.30 15.84,17.57 16.3,18.03 C8.1 B1.VCC

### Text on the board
tPlace: Squall | A
bPlace: Brad / Campbell | 2014/10/08

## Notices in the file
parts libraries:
SparkFun-LED: Licensing: CC v3.0 Share-Alike You are welcome to use this library for commercial purposes.
